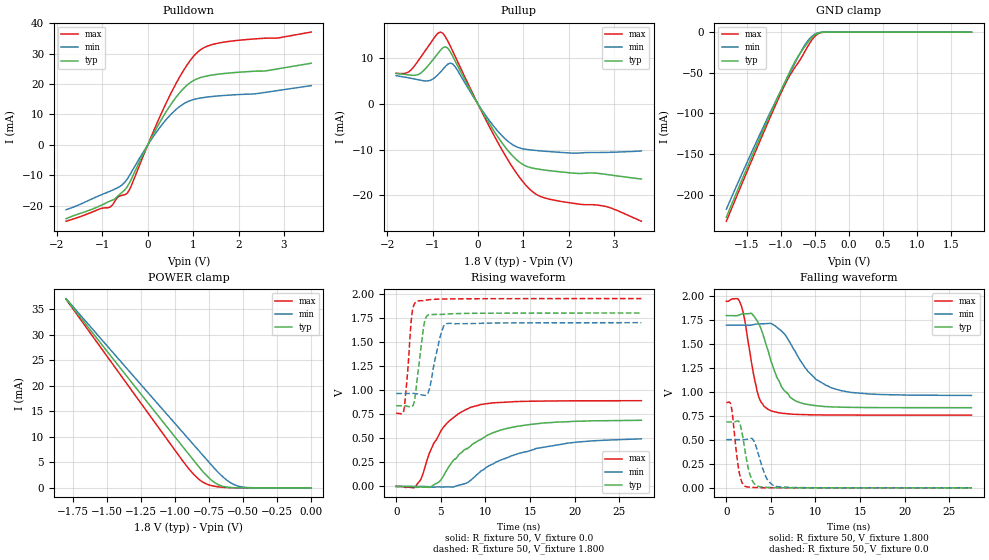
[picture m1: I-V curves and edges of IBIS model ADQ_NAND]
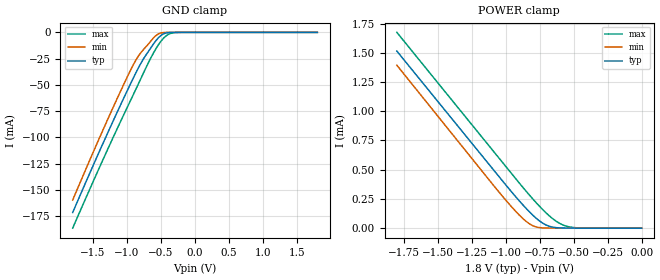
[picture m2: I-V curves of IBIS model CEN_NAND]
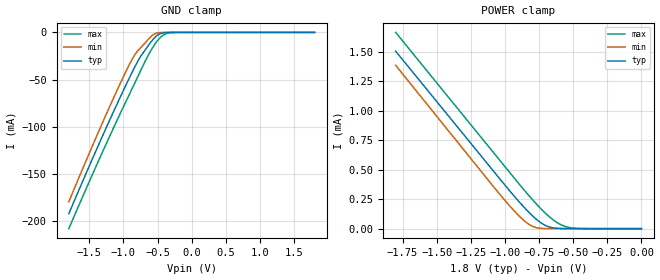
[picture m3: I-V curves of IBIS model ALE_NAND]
| This IBIS file was created by s2ibis3 version 1.1
| North Carolina State University, ERL, 2006
[IBIS ver] 3.2
[File name] s34ms02g1_b_i_18_r2.ibs
[File Rev] 2.0
|   Rev1.0 Initial release with updated measurement
|   (X16 ONFI F41 98798AE 41087)
|   Rev2.0 Update 0A for 0V
[Date] 7/23/2014
[Source] Spansion IBIS team
|   Email: dl.ibisteam@spansion.com
[Notes]  Generated IBIS models from SPICE simulations.
|   VIO=1.65V - 1.95V, Temperature Range: Industrial (-30oC to +85oC).
[Disclaimer] THE MODEL LIBRARIES ARE PROVIDED AS IS.
[Copyright] (C) COPYRIGHT 2014
| SPANSION LLC
| ALL RIGHTS RESERVED.
|   Component S34MS02G1 X16 ONFI F41 in VBM063 package
[Component]   S34MS02G1
[Manufacturer]   Spansion
[Package]
| variable   typ   min   max
R_pkg   153.52mOhm   132.26mOhm   175.35mOhm
L_pkg   3.70nH   2.89nH   4.77nH
C_pkg   1.24pF   1.06pF   1.56pF
[Pin]   signal_name   model_name   R_pin   L_pin   C_pin
A1   R   NC
A2   R   NC
A9   R   NC
A10   R   NC
B1   R   NC
B9   R   NC
B10   R   NC
C3   WP#   WP_NAND   175.35m   4.59n   1.56p
C4   ALE   ALE_NAND   170.69m   4.5n   1.4p
C5   VSS   GND
C6   CE#   CEN_NAND   142.25m   3.23n   1.11p
C7   WE#   WEN_NAND   162.28m   3.8n   1.32p
C8   RB#   RB_NAND   132.26m   3.01n   1.14p
D3   VDD   POWER
D4   RE#   REN_NAND   155.95m   4.22n   1.36p
D5   CLE   CLE_NAND   146.15m   3.48n   1.2p
D6   R   NC
D7   R   NC
D8   R   NC
E3   R   NC
E4   R   NC
E5   R   NC
E6   R   NC
E7   R   NC
E8   R   NC
F3   R   NC
F4   R   NC
F5   R   NC
F6   R   NC
F7   VSS   GND
F8   R   NC
G3   R   NC
G4   VDD   POWER
G5   R   NC
G6   I/O13   ADQ_NAND   143.41m   2.99n   1.09p
G7   I/O15   ADQ_NAND   147.26m   2.89n   1.14p
G8   R   NC
H3   I/O8   ADQ_NAND   164.9m   4.77n   1.39p
H4   I/O0   ADQ_NAND   160.59m   3.98n   1.35p
H5   I/O10   ADQ_NAND   137.07m   3.5n   1.06p
H6   I/O12   ADQ_NAND   149.88m   3.02n   1.14p
H7   I/O14   ADQ_NAND   143.43m   3n   1.12p
H8   VDD   POWER
J3   I/O9   ADQ_NAND   163.61m   4.74n   1.37p
J4   I/O1   ADQ_NAND   156.39m   4.36n   1.28p
J5   I/O11   ADQ_NAND   147.34m   3.53n   1.11p
J6   VDD   POWER
J7   I/O5   ADQ_NAND   147.09m   3.27n   1.16p
J8   I/O7   ADQ_NAND   151.06m   3.34n   1.14p
K3   VSS   GND
K4   I/O2   ADQ_NAND   163.82m   4.01n   1.29p
K5   I/O3   ADQ_NAND   149.37m   3.59n   1.11p
K6   I/O4   ADQ_NAND   160.31m   3.6n   1.29p
K7   I/O6   ADQ_NAND   160.51m   3.73n   1.28p
K8   VSS   GND
L1   R   NC
L2   R   NC
L9   R   NC
L10   R   NC
M1   R   NC
M2   R   NC
M9   R   NC
M10   R   NC
| Models and submodels in the file (8): ADQ_NAND (I/O), CEN_NAND (Input), ALE_NAND (Input), CLE_NAND (Input), WEN_NAND (Input), REN_NAND (Input), WP_NAND (Input), RB_NAND (Open_drain)
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|   Model ADQ_NAND
[Model]   ADQ_NAND
Model_type   I/O
Polarity   Non-Inverting
Enable   Active-High
Vinl   = 0.360V
Vinh   = 1.440V
Vmeas  = 0.900V
Vref   = 0.900V
Rref   = 8350ohm
Cref   = 30pF
| variable   typ   min   max
C_comp   3.72pF   3.35pF   4.46pF
| variable   typ   min   max
[Temperature Range]  25.00   85.00   -30.00
[Voltage Range]   1.800   1.700   1.950
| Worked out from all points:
|   slope of the pulldown table from 0 to 0.27 V, typ, clamps not added: 35.8 ohm
|   slope of the pullup table from 0 to 0.27 V, typ, clamps not added: 58.9 ohm
|   GND clamp passes 1 mA (typ) near -0.44 V on its own axis
|   POWER clamp passes 1 mA (typ) near -0.71 V on its own axis
|   rising waveform, R_fixture 50, V_fixture 0.0: 20-80 % time 5.18ns typ, 7.01ns min, 3.23ns max; typ from 0 V to 0.687 V
|   falling waveform, R_fixture 50, V_fixture 1.800: 20-80 % time 2.28ns typ, 3.54ns min, 1.35ns max; typ from 1.8 V to 0.838 V
|   rising waveform, R_fixture 50, V_fixture 1.800: 20-80 % time 754ps typ, 979ps min, 578ps max; typ from 0.838 V to 1.8 V
|   falling waveform, R_fixture 50, V_fixture 0.0: 20-80 % time 849ps typ, 1.08ns min, 665ps max; typ from 0.688 V to 0 V
[Pulldown]
| voltage   I(typ)   I(min)   I(max)
-1.8V     -24.24mA   -21.3mA    -25.1mA
-828mV    -18.44mA   -15.22mA   -20.42mA
-666mV    -16.9mA    -14.08mA   -17.25mA
-450mV    -13.69mA   -11.16mA   -15.84mA
-342mV    -10.59mA   -8.492mA   -12.67mA
90mV      2.627mA    2.052mA    3.223mA
468mV     12.38mA    9.368mA    15.7mA
792mV     18.59mA    13.51mA    24.57mA
1.116V    21.88mA    15.27mA    30.73mA
1.602V    23.31mA    16.14mA    33.56mA
2.628V    24.38mA    17.33mA    35.06mA
3.6V      26.82mA    19.46mA    37.06mA
[Pullup]
| voltage   I(typ)   I(min)   I(max)
-1.8V     6.711mA    6.204mA    6.703mA
-1.53V    6.378mA    5.733mA    7.009mA
-1.314V   6.462mA    5.32mA     9.487mA
-1.044V   9.028mA    5.211mA    13.32mA
-774mV    12.29mA    7.564mA    15.5mA
-558mV    10.5mA     8.79mA     11.62mA
468mV     -7.609mA   -6.274mA   -8.926mA
792mV     -11.62mA   -9.059mA   -14.28mA
1.116V    -13.78mA   -9.986mA   -18.39mA
1.494V    -14.47mA   -10.34mA   -20.6mA
2.844V    -15.42mA   -10.57mA   -22.48mA
3.6V      -16.4mA    -10.26mA   -25.64mA
[GND_clamp]
| voltage   I(typ)   I(min)   I(max)
-1.8V     -227.8mA   -218mA     -232.8mA
-1.44V    -155.9mA   -150mA     -160.5mA
-1.152V   -100.6mA   -98.3mA    -104.1mA
-972mV    -67.31mA   -67.55mA   -70.33mA
-864mV    -48.19mA   -49.77mA   -52.81mA
-756mV    -31.2mA    -32.3mA    -39.05mA
-612mV    -13.69mA   -11.59mA   -18.85mA
-540mV    -6.376mA   -4.919mA   -9.319mA
-468mV    -1.892mA   -1.445mA   -2.895mA
-396mV    -317.5uA   -280.6uA   -453uA
-324mV    -33.8uA    -40.79uA   -36.53uA
1.8V      190.5pA    3.644nA    114.8pA
[POWER_clamp]
| voltage   I(typ)   I(min)   I(max)
-1.8V     36.95mA    37.04mA    36.91mA
-936mV    7.811mA    10.64mA    5.005mA
-864mV    5.405mA    8.449mA    2.668mA
-810mV    3.633mA    6.808mA    1.367mA
-738mV    1.629mA    4.621mA    470.5uA
-684mV    632.8uA    3.05mA     201.6uA
-612mV    108.6uA    1.346mA    45.35uA
-540mV    13.14uA    364uA      4.716uA
-432mV    393.1nA    23.68uA    63.01nA
0V        0A         0A         0A
[Ramp]
| variable   typ   min   max
dV/dt_r   412.33m/5.13n   297.56m/6.78n   534.08m/3.12n
dV/dt_f   577.47m/2.21n   440.84m/3.34n   713.83m/1.33n
R_load = 50
[Rising Waveform]
R_fixture = 50
V_fixture = 0.0
| time   V(typ)   V(min)   V(max)
0s        35.16uV    -178.1nV   566.9uV
2.14ns    -6.557mV   130.9uV    -3.442mV
2.788ns   -6.033mV   243.2uV    79.41mV
3.724ns   -9.674mV   -3.583mV   345.6mV
5.02ns    69.11mV    -5.603mV   578.2mV
6.388ns   268.6mV    -6.468mV   712.1mV
8.224ns   410.3mV    54.63mV    818.5mV
11.14ns   567mV      250.5mV    869.2mV
15.57ns   649.1mV    391.9mV    885.1mV
27.5ns    686.7mV    494.2mV    890.1mV
[Falling Waveform]
R_fixture   = 50
V_fixture   = 1.800
V_fixture_min = 1.700
V_fixture_max = 1.950
| time   V(typ)   V(min)   V(max)
0s        1.8V       1.7V       1.949V
1.636ns   1.814V     1.7V       1.915V
2.788ns   1.823V     1.701V     1.33V
3.508ns   1.738V     1.713V     991.1mV
4.804ns   1.395V     1.718V     813.9mV
6.136ns   1.063V     1.643V     780.5mV
7.108ns   950.1mV    1.523V     772mV
9.124ns   870.7mV    1.22V      764mV
11.61ns   846.8mV    1.052V     761.3mV
27.5ns    837.6mV    965.4mV    760.3mV
[Rising Waveform]
R_fixture   = 50
V_fixture   = 1.800
V_fixture_min = 1.700
V_fixture_max = 1.950
| time   V(typ)   V(min)   V(max)
0s        837.5mV    965.1mV    760.9mV
880ps     837.4mV    965.1mV    802.3mV
1.744ns   827.2mV    966mV      1.774V
2.068ns   900.2mV    964.8mV    1.901V
2.356ns   1.119V     961.3mV    1.923V
3.328ns   1.752V     947.4mV    1.934V
3.76ns    1.784V     1.024V     1.939V
5.02ns    1.785V     1.582V     1.945V
5.632ns   1.789V     1.689V     1.946V
27.5ns    1.8V       1.7V       1.95V
[Falling Waveform]
R_fixture = 50
V_fixture = 0.0
| time   V(typ)   V(min)   V(max)
0s        688.2mV    503.8mV    890.1mV
556ps     688mV      503.8mV    846.1mV
1.42ns    690.5mV    503.7mV    174.4mV
1.744ns   583.4mV    503.6mV    58.33mV
2.176ns   344.4mV    505.6mV    13.62mV
2.572ns   163.6mV    514.1mV    7.024mV
3.112ns   45.85mV    484.8mV    3.77mV
4.48ns    5.218mV    106.9mV    1.058mV
5.56ns    2.061mV    15.63mV    502.1uV
27.5ns    -1.069uV   450.8nV    -607.7nV
|   Model CEN_NAND
[Model]   CEN_NAND
Model_type   Input
Vinl = 0.360V
Vinh = 1.440V
| variable   typ   min   max
C_comp   2.20pF   1.98pF   2.64pF
| variable   typ   min   max
[Temperature Range]  25.00   -30.00   85.00
[Voltage Range]   1.800   1.700   1.950
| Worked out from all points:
|   GND clamp passes 1 mA (typ) near -0.44 V on its own axis
|   POWER clamp passes 1 mA (typ) near -1.44 V on its own axis
[GND_clamp]
| voltage   I(typ)   I(min)   I(max)
-1.8V     -171.6mA   -159.8mA   -186.5mA
-1.296V   -97.42mA   -84.54mA   -113mA
-1.044V   -62mA      -48.92mA   -77.85mA
-900mV    -42.52mA   -29.89mA   -58.24mA
-828mV    -33.22mA   -22.07mA   -48.35mA
-756mV    -24.99mA   -16.18mA   -38.4mA
-612mV    -11.15mA   -5.36mA    -19.76mA
-504mV    -3.085mA   -583.3uA   -8.654mA
-432mV    -700.3uA   -55.3uA    -3.629mA
-360mV    -93.93uA   -2.943uA   -1.015mA
-252mV    -2.155uA   -17.44nA   -71.47uA
1.8V      140.8pA    79.49pA    15.92nA
[POWER_clamp]
| voltage   I(typ)   I(min)   I(max)
-1.8V     1.514mA    1.393mA    1.674mA
-1.026V   408.5uA    277uA      566.8uA
-900mV    234.3uA    112.6uA    386.8uA
-828mV    143.4uA    39.7uA     287.2uA
-774mV    83.73uA    9.844uA    216.3uA
-702mV    26.55uA    788.6nA    130.1uA
-630mV    4.495uA    62.15nA    60.75uA
-558mV    538.1nA    3.703nA    18.71uA
-450mV    16.7nA     132.3pA    1.525uA
0V        0A         0A         0A
|   Model ALE_NAND
[Model]   ALE_NAND
Model_type   Input
Vinl = 0.360V
Vinh = 1.440V
| variable   typ   min   max
C_comp   2.20pF   1.98pF   2.64pF
| variable   typ   min   max
[Temperature Range]  25.00   -30.00   85.00
[Voltage Range]   1.800   1.700   1.950
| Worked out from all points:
|   GND clamp passes 1 mA (typ) near -0.44 V on its own axis
|   POWER clamp passes 1 mA (typ) near -1.44 V on its own axis
[GND_clamp]
| voltage   I(typ)   I(min)   I(max)
-1.8V     -192.3mA   -179.6mA   -208.1mA
-1.26V    -102.4mA   -88.17mA   -119.4mA
-1.008V   -62.69mA   -48.22mA   -80.06mA
-864mV    -41.05mA   -27.42mA   -58.29mA
-756mV    -26.47mA   -16.77mA   -41.79mA
-648mV    -15.24mA   -8.416mA   -25.81mA
-576mV    -8.287mA   -3.156mA   -16.52mA
-504mV    -3.152mA   -587.1uA   -8.981mA
-432mV    -704.7uA   -55.34uA   -3.704mA
-360mV    -94.01uA   -2.944uA   -1.022mA
-252mV    -2.155uA   -17.44nA   -71.51uA
1.8V      140.8pA    79.49pA    15.92nA
[POWER_clamp]
| voltage   I(typ)   I(min)   I(max)
-1.8V     1.507mA    1.387mA    1.667mA
-1.026V   406.6uA    275.7uA    564.2uA
-900mV    233.3uA    112.2uA    385.1uA
-828mV    142.8uA    39.6uA     285.9uA
-774mV    83.46uA    9.834uA    215.4uA
-702mV    26.5uA     788.5nA    129.7uA
-630mV    4.493uA    62.15nA    60.59uA
-558mV    538.1nA    3.703nA    18.69uA
-450mV    16.7nA     132.3pA    1.525uA
0V        0A         0A         0A
